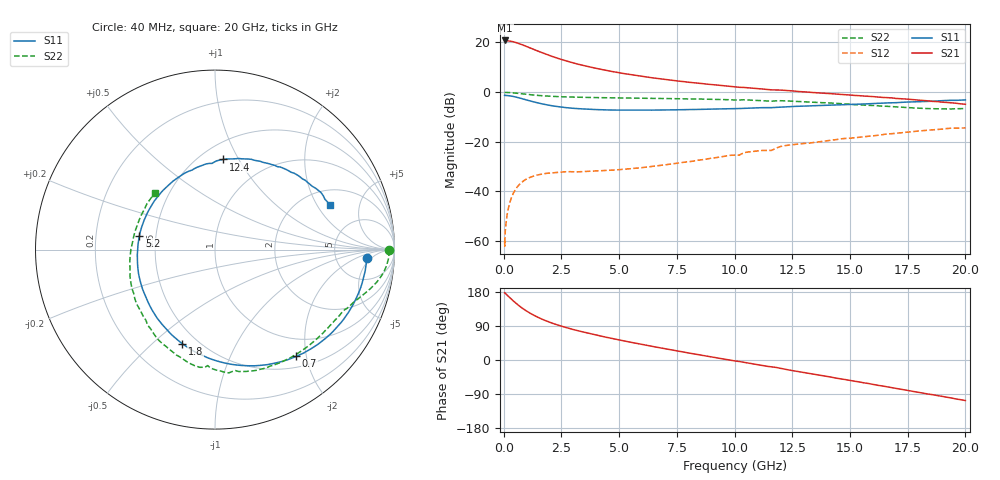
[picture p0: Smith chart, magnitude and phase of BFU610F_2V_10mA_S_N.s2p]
! Filename:  P:\Prog\Test\Noise\ATS_data\Testdata_Net\SplitFiles\BFU610_2W_A5_HighFreq_2V_10mA_D.s2p
! Date/Time: Wed 10/Aug/2011 16:56:16
! BFU610_2W_A5_HighFreq_2V_1mA_10mA_Bias7_R.s2p
! MDIF S-parameter v. bias file
! BFU610_2W_A5_HighFreq_2V_1mA_10mA
! Date/time Mon Aug 08 14:20:39 2011
! VAR V_out= 2.0002
! VAR I_out= 9.9950
! VAR V_in= 0.9342
! VAR I_in= 0.0972
! Device data file deembeded for feedlines and parallel
! Original file: \SplitFiles\BFU610_2W_A5_HighFreq_2V_10mA_R.s2p
! Feed-files: PR003V01_101208_Feed1.s2p, PR003V01_101208_Feed2.s2p
! Parallel-file: PR003V01_101208_Par.s2p
# MHz S MA R 50
!  Freq-MHz  S11-mag  S11-arg  S21-mag  S21-arg  S12-mag  S12-arg  S22-mag  S22-arg
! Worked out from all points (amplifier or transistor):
!   167 points, 40 MHz to 20 GHz, reference 50 ohm
!   highest |S21| = 20.6 dB at 60 MHz (marker M1)
!   |S21| within 3 dB of that: start of sweep to 1.144 GHz
!   unconditionally stable (mu >= 1): start of sweep to 51.49 MHz; 2.021 GHz to end of sweep
!   at 550 MHz: K = 0.31, MSG = 29.2 dB, |S12| = -38.7 dB
!   at 4.2 GHz: K = 2.16, MAG = 14.3 dB, |S12| = -31.7 dB
!   at 20 GHz: K = 1.92, MAG = -0.8 dB, |S12| = -14.5 dB
!   lowest NFmin = 1.67 dB at 400 MHz
!   S11 on the Smith chart (normalised r, x): 40 MHz: 11, -4; 700 MHz: 0.68, -1.82; 1.8 GHz: 0.41, -0.63; 5.2 GHz: 0.40, +0.08; 12.4 GHz: 0.64, +0.87; 20 GHz: 2.75, +2.60
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40  0.8466 -3.2  10.71 177.5  0.000991 76.4  0.9678 -0.2
50  0.8396 -4.3  10.67 177.3  0.0007983 84.5  0.9684 -0.5
60  0.846 -4.5  10.71 176.2  0.001386 88.3  0.9696 -0.7
220  0.8345 -17.6  10.52 167.0  0.004999 79.2  0.9651 -3.9
400  0.8076 -31.5  10.11 156.8  0.008838 72.2  0.9516 -7.0
550  0.7797 -42.5  9.665 148.8  0.01166 66.5  0.9362 -9.3
700  0.7475 -52.7  9.141 141.6  0.0141 61.1  0.9197 -11.3
950  0.6936 -68.4  8.245 130.8  0.01733 53.5  0.8923 -14.2
1250  0.6357 -84.7  7.236 119.9  0.02005 46.4  0.8632 -16.9
1500  0.594 -96.6  6.503 112.2  0.02162 41.9  0.844 -18.9
1800  0.5554 -109.1  5.752 104.2  0.02287 37.8  0.8251 -21.0
2100  0.5227 -120.2  5.12 97.2  0.02366 34.8  0.8108 -23.1
2500  0.4926 -133.0  4.446 89.3  0.0245 32.5  0.7931 -25.6
3400  0.4534 -156.1  3.413 74.5  0.02495 31.0  0.7732 -31.4
4200  0.4359 -172.8  2.829 63.2  0.02606 32.6  0.7613 -36.8
5200  0.4284 169.8  2.322 50.6  0.02781 36.6  0.7501 -43.8
6800  0.4303 146.3  1.813 31.9  0.03333 42.8  0.7338 -55.5
10200  0.461 106.0  1.231 -3.9  0.05347 47.5  0.6842 -81.2
12400  0.5047 84.6  1.048 -26.9  0.08565 39.0  0.6502 -102.2
13400  0.5247 75.4  0.9654 -37.0  0.09559 32.5  0.6165 -112.6
16800  0.6012 46.9  0.7551 -72.9  0.1441 8.7  0.5042 -158.3
20000  0.6864 21.3  0.5615 -107.0  0.1886 -23.6  0.4602 136.8
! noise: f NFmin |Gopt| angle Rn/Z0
400  1.674  0.3683  3.58  0.4193
700  1.789  0.3381  6.136  0.4282
1150  1.967  0.2934  9.893  0.4363
1600  2.152  0.2494  13.57  0.4395
2050  2.342  0.2061  17.2  0.4393
2600  2.584  0.1545  21.57  0.4368
3500  3  0.07363  28.44  0.4344
4400  3.441  0.00218  268.7  0.4449
5600  4.069  0.08992  231.1  0.5004
8000  5.46  0.2382  263.8  0.8643
